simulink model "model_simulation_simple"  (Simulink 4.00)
settings: Solver=VariableStepDiscrete  StartTime=0.0  StopTime=ts  RelTol=1e-3
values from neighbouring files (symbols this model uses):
  A = [0.9944 -0.1203 -0.4302    [model_simple.m]
  Ao = A - K * C    [model_simple.m]
  B = [0.4252 -0.0082 0.1813]'    [model_simple.m]
  Bo = [B K]    [model_simple.m]
  C = [1 0 0]    [model_simple.m]
  Co = C    [model_simple.m]
  D = 0    [model_simple.m]
  Do = zeros(1,2)    [model_simple.m]
  Tc = 0.1    [model_simple.m]
  tfy = ts/2    (= 25)    [model_simple.m]
  x0 = [0.05 0.15 0.2]    [model_simple.m]

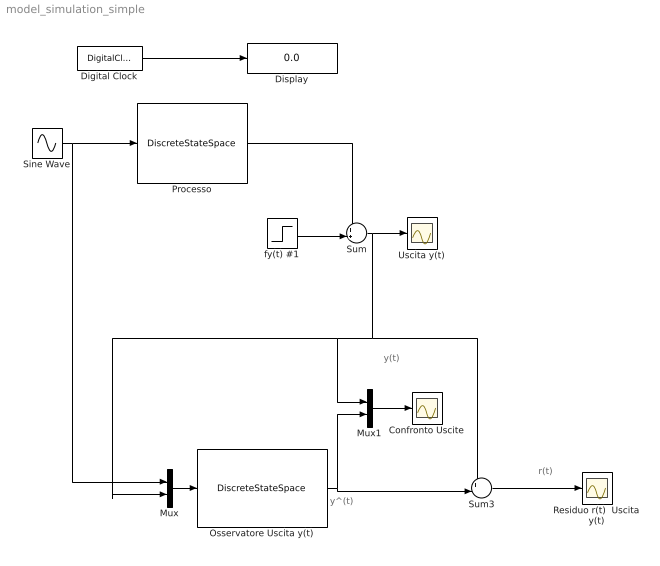
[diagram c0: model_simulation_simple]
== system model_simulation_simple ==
  note: y(t)
  note: y^(t)
  note: r(t)
  Confronto Uscite : Scope
  Digital Clock : DigitalClock  SampleTime=Tc
  Display : Display
  Mux : Mux  Inputs=2
  Mux1 : Mux  Inputs=2
  Osservatore Uscita y(t) : DiscreteStateSpace  A=Ao  B=Bo  C=Co  D=Do  X0=0  SampleTime=Tc  Realization=auto
  Processo : DiscreteStateSpace  A=A  B=B  C=C  D=D  X0=x0  SampleTime=Tc  Realization=auto
  Residuo r(t)  Uscita y(t) : Scope
  Sine Wave : Sin  SineType=Time-based  Amplitude=1  Bias=0  Frequency=1  Phase=0  Samples=10  SampleTime=Tc
  Sum : Sum  Inputs=++|  SaturateOnIntegerOverflow=on
  Sum3 : Sum  Inputs=+-|  SaturateOnIntegerOverflow=on
  Uscita y(t) : Scope
  fy(t) #1 : Step  Time=tfy  Before=0  After=1  SampleTime=Tc
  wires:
  Sine Wave/1 -> Processo/1, Mux/1
  Processo/1 -> Sum/1
  Osservatore Uscita y(t)/1 -> Sum3/2, Mux1/2
  Mux/1 -> Osservatore Uscita y(t)/1
  Digital Clock/1 -> Display/1
  Sum/1 -> Uscita y(t)/1, Sum3/1, Mux/2, Mux1/1
  fy(t) #1/1 -> Sum/2
  Sum3/1 -> Residuo r(t)  Uscita y(t)/1
  Mux1/1 -> Confronto Uscite/1
